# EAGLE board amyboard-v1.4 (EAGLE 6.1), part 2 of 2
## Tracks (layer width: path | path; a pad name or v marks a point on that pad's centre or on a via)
3V3_IN  (via drill 0.3)
  Top 0.61: D2.A 74.28,43.91 R59.1 74.3,45.99 v74.3,47.65 73.25,48.69 TP7.T | I2C_CONTROL.3 79.61,47.65 v79.43,47.65
  Top 0.813: Q3.2 74.96,44.59 D2.A
  Bottom 0.61: v79.43,47.65 v74.3,47.65
5V_IN
  Top 0.305: C34.2 C85.2 62.37,46.09 FB3.2 63.96,43.95 D14.A | C34.2 60.83,44.67 D3.A | C52.2 C34.2
  Top 0.406: R58.1 59.5,45.25 59.69,45.44
  Top 0.61: TP8.T 58.98,46.15 59.69,45.44
  pour Top: 59.28,46.43 64.77,46.43 64.77,42.83 60.76,42.83 59.46,44.12 59.28,44.3
12_IN  (via drill 0.3)
  Top 0.406: D1.A 68.58,40.82 | 68.58,40.82 D4.A | 68.1,39.83 69.14,39.83 | 69.62,40.29 69.62,39.83 69.14,39.83 | 69.14,39.83 v69.11,40.41 | 68.61,40.29 68.61,40.79 68.58,40.82 | 69.7,20.68 69,20.68 R57.1
  Top 0.61: v57.05,27.53 57.05,15.27 58.14,14.17 68.22,14.17 | P1.5 68.99,13.59 68.4,14.17 | 68.4,14.17 68.22,14.17 | 69.01,14.96 68.22,14.17 | 68.4,14.17 68.99,14.17
  Top 0.813: 69.62,40.29 68.61,40.29 | D1.A 68.83,41.58 69.77,41.58 69.22,41.02 68.58,41.02 | P1.5 68.99,14.17 P1.6 68.99,19.97 69.7,20.68 TP9.T
  Bottom 0.61: v69.11,40.41 61.72,40.41 60.81,39.5 60.81,37.52 55.93,32.64 55.93,28.65 v57.05,27.53
12V5_UNREG  (1 unrouted)
  Top 0.254: 59.33,29.57 59.82,30.05 60.25,29.62 61.09,29.62
  Top 0.406: U8.1 57.9,29.93 58.27,29.57 59.33,29.57 59.94,29.57 | 59.94,29.57 61.17,29.57 | U8.3 59.8,29.71 59.94,29.57
  Top 0.61: C18.1 61.87,28.98 R15.1
13.5V  (via drill 0.3)  (1 unrouted)
  Top 0.305: R15.2 61.32,31.27 61.29,31.29 | 62.28,31.29 62,31.57 62,31.85 62,31.88 62.08,31.95 | 62.47,31.41 62.45,31.41 62.18,31.67
  Top 0.406: v50.09,36.5 58.04,36.5 C29.1 58.84,35.7 R19.1 | R19.1 R16.1 61.06,33.64 D8.C | C20.2 59.94,34.76 R19.1 | C19.1 62.47,31.41 | 58.75,35.87 58.75,35.84 58.9,35.69 59.36,35.69 59.74,35.31 59.74,34.52 60.35,34.52 61.21,33.66 | 61.21,31.29 61.29,31.29 62.28,31.29 | 61.62,31.95 61.62,31.88 | 62,31.85 62,34.29 61.21,35.08 61.21,35.81 59.46,35.81 59.13,36.15 59.05,36.15 | 58.62,36.15 59.05,36.15 | 59.05,36.15 59.66,35.54 60.5,35.54 61.62,34.42 61.19,34.42 60.27,35.33 60.27,34.85 60.76,34.37 | U3.5 39.26,31.19 39.65,31.57 40.5,31.57 C26.2 40.58,31.62 v41.22,31.62
  Top 0.61: 61.21,33.66 61.21,31.29 | 62.18,31.95 62.08,31.95 61.62,31.95 | 61.62,31.88 61.82,31.67 62.18,31.67
  Bottom 0.406: v50.09,36.5 49.25,36.5 44.37,31.62 v41.22,31.62
+3V3  (via drill 0.3)  (3 unrouted)
  Top 0.254: C5.1 U1.22 27.33,26.57 26.42,27.48 | R54.1 R34.1 4.7,18.89 v4.7,19.43 | C33.2 R43.2 | 25.17,29.24 U1.36 25.42,29.05 | 25.17,29.24 25.17,31.17 24.8,31.54 | 25.4,28.7 24.99,29.11 | 24.99,29.11 24.99,29.36 | 24.99,29.36 24.99,30.48 | 24.33,31.34 24.77,31.34 24.99,31.12 24.99,30.48 | 26.42,27.48 26.34,27.56 25.53,27.56 24.99,28.09 24.99,29.11 | 24.99,29.36 25.16,29.2 | 25.16,29.2 25.2,29.16 25.2,28.17 25.68,27.69 26.34,27.69 26.36,27.71 26.36,27.81 | 26.36,27.81 26.31,27.76 25.65,27.76 25.43,27.99 25.43,28.5 | 24.99,30.48 v25.04,30.43 | C40.1 40.26,19.14 40.26,19.66 | C15.1 26.42,31.2 U1.34 26.42,27.48 | 39.27,22.63 39.32,22.68 40.66,22.68 40.82,22.53 40.82,19.33 40.39,18.9 39.42,18.9 39.19,19.13 | 40.56,21.01 40.64,21.08 v40.64,21.39 | 39.29,20.5 39.24,20.55 PCM5101.20 | v27.33,22.63 | 26.42,27.92 26.42,27.81 | 26.42,27.81 27.56,26.67 30.86,26.67 30.96,26.57 30.81,26.42 27.76,26.42 27.56,26.21 26.19,27.59 25.86,27.59 | 26.36,27.81 26.42,27.81 | 25.38,29.01 25.42,29.05 | 25.09,30.61 25.43,30.28 25.43,29.06 25.42,29.05 | 25.17,29.24 25.17,29.21 25.16,29.2 | C3.+ 38.75,19.16 38.99,18.92 | 86.21,35.21 86.41,35.21 C39.2
  Top 0.305: D12.4 R44.2 R42.2 R43.2 | 38.38,19.03 38.89,19.03 38.99,18.92 40.34,18.92 40.46,19.05 40.46,20.91 | 40.46,20.91 40.56,21.01 40.56,22.43 40.34,22.65 PCM5101.17 39.38,22.65 | 40.46,20.91 40.28,20.73 38.68,20.73 38.66,20.7 38.66,19.86 38.23,19.43 38.63,19.43 39.73,20.52 38.91,20.52 38.86,20.47 38.86,20.07 | 38.86,19.81 38.86,20.07 | 38.86,20.07 39.29,20.5 39.75,20.5 40.26,19.99 40.26,19.66 39.67,19.08 40.01,19.08 40.21,19.28
  Top 0.406: R35.1 14.02,15.04 | 14.02,15.04 C35.1 14.38,15.3 14.38,15.39 | U15.6 14.38,15.39 | 14.02,15.04 14.38,15.39 | v86.91,44.58 86.79,44.69 R41.2 82.49,44.69 L1.P$2 | R39.2 86.91,46.59 C27.1 87.4,46.84 89.08,48.51 92.43,48.51 93.04,49.12 93.04,51.77 91.77,53.04 89.72,53.04 R68.2 89.18,53 | D12.4 85.61,41.06 | 89.18,53 88.7,53 R69.2 | TP1.T 89.18,53.47 | 89.18,53.47 89.18,53 | 88.75,53.01 88.75,53.04 89.18,53.47 | 89.18,53.47 89.2,53.47 89.64,53.04
  Top 0.508: R40.2 v86.91,44.58 R39.2 | 97.16,33.78 97.16,34.71 R47.2
  Top 0.61: C37.2 96.84,35.03 R47.2 | C38.1 97.21,33.83 97.16,33.78 | R55.1 v84.18,33.78 84.78,33.78 | 84.18,42.49 82.25,42.49 82.02,42.72 L1.P$2 | 21.64,33.97 T1.4 v21.64,32.14 v21.64,32.13 | 84.78,33.78 84.99,33.78 C39.2 86.26,35.26 86.21,35.21 84.78,33.78 | U15.6 v14.38,22.1 | R49.2 77.75,20.07 76.02,21.79 HOST.1 | 39.19,19.13 39.19,19.51 40.11,20.42 40.11,19.84 39.47,19.2 40.13,19.2 40.54,19.61 40.54,20.7 40.72,20.88 | 40.72,20.88 40.72,22.38 | 40.72,20.88 40.72,19.48 40.34,19.1 | 27.33,26.57 v27.33,22.63
  Top 0.813: SD1.4 95.11,42.55 97.16,40.51 97.16,33.78 U2.2 | SD1.4 92.28,42.55 | Q3.3 84.18,42.49 | 84.18,42.49 85.61,41.06 86.21,40.46 86.21,35.21 | 79.35,42.5 80.09,43.23 83.82,43.23 83.82,42.85 84.18,42.5 | 84.18,42.49 84.18,42.5 | 84.18,42.5 84.18,44.15 84.81,44.78 86.39,44.78 86.82,44.35 86.82,46.46 86.67,46.31 86.67,46.05 85.65,45.04 83.82,45.04 83.03,44.25 83.84,44.25 84.45,44.86 86.11,44.86 86.59,45.34 | SD1.4 89.98,42.55 v89.97,42.57 | T1.1 T1.4
  Bottom 0.254: I2C_HOST.3 5.22,19.95 v4.7,19.43
  Bottom 0.61: v25.04,30.43 23.34,30.43 v21.64,32.13 | v84.18,33.78 84.18,23.9 82.6,22.33 HOST.1 74.45,22.33 73.2,21.08 53.65,21.08 53.16,20.6 41.43,20.6 39.4,22.63 v27.33,22.63 26.8,22.1 v14.38,22.1 10.31,22.1 8.15,19.94 5.8,19.94 I2C_HOST.3
  Bottom 0.813: v86.91,44.58 89.08,44.58 89.97,43.69 v89.97,42.57
-12.6V
  Top 0.61: D10.A 69.73,29.46 C31.2 67.61,29.46 67.41,29.67 | R17.2 67.41,29.67 | 67.41,29.67 C25.1
A3V3  (via drill 0.3)  (2 unrouted)
  Top 0.254: U5.8 2.41,21.54 v2.29,21.67 | C22.+ 42.78,26.31 v42.85,26.24 | U1.42 22.25,25.07 21.03,26.29 20.87,26.29 C11.1
  Top 0.305: R31.1 3.12,28.68 v3.57,29.12 4.01,29.57 4.01,30.2 4.06,30.25 4.06,30.18 4.04,30.15 4.04,31.27 4.01,31.29
  Top 0.406: 4.06,30.16 R20.2 | 42.85,25.15 42.85,24.77 43.33,25.25 43.26,25.25 42.88,25.63 | 42.85,25.15 42.85,28.66 C22.+ 42.67,28.21 42.67,21.13 43.11,20.7 PCM5101.1 45.79,20.7 C46.1 47.86,19.8 C45.+ 48.15,19.76 TP2.T | 42.85,25.15 42.95,25.25 PCM5101.8 47.23,25.25 C47.1 R13.2 R12.2 | 19.48,26.4 20.1,26.4 v20.17,26.47 | v61.01,24.69 61.01,24.14 R23.1 61,23.08 C54.1 61.02,23.1 U10.1
  Top 0.61: C11.1 19.48,26.4 C12.+
  Bottom 0.406: 20.17,26.65 v20.17,26.47 19.99,26.65 | 20.17,26.65 20.4,26.65 | 20.4,26.65 42.44,26.65 v42.85,26.24 44.4,24.69 v61.01,24.69 | 3.94,26.65 3.67,26.65 3.57,26.75 v3.57,29.12 3.57,22.95 v2.29,21.67 | 3.94,26.65 19.94,26.65 | 19.94,26.65 19.99,26.65 | 19.99,26.65 20.17,26.65 | 3.58,27 3.94,26.65 | 3.94,26.65 3.58,26.29 | 20.4,26.65 20.17,26.42 19.94,26.65
A5V  (via drill 0.3)
  Top 0.254: C16.+ 21.96,21.21 C13.1 22.52,23.07 U1.46 v26.04,23.06
  Top 0.61: U9.1 TP3.T C53.1 v72.64,21.9
  Bottom 0.254: v72.64,21.9 53.34,21.9 52.78,21.34 41.81,21.34 39.83,23.32 26.29,23.32 v26.04,23.06
A12V  (via drill 0.3)
  Top 0.406: U4.4 v49.07,31.85 | C32.1 57.28,33.38 | 57.28,33.38 57.8,33.38 U8.5 | v57.3,32.72 57.3,33.35 57.28,33.38 | 56.34,33.4 56.62,33.4 v57.3,32.72 | v57.3,32.72 57.58,33 57.96,33
  Top 0.61: TP4.T 45.85,31.85 U4.4 | U10.3 66.27,23.88 66.27,25.58 | 66.27,25.58 v66.27,26.44 v66.28,26.44 U9.3 | 67.54,26.37 67.54,26.01 66.7,26.01 66.27,25.58
  Bottom 0.406: v49.07,31.85 49.07,28.93 51.59,26.42 57.45,26.42 | 57.45,26.42 57.99,26.42 | 57.99,26.42 58.52,26.42 | 58.52,26.42 66.24,26.42 v66.27,26.44 | v57.3,32.72 57.3,28.65 57.99,27.97 57.99,26.95 | 57.99,26.95 57.99,26.42 | 57.45,26.42 57.99,26.95 | 57.99,26.95 58.52,26.42
A-12V
  Top 0.406: 56.79,30.35 56.74,30.4 56.74,30.43 TP5.T 56.6,30.34 56.43,30.34 | 57.93,28.81 U7.5 57.93,28.84 56.43,30.34 | U4.11 53.72,31.85 54.28,31.29 C28.1 55.47,31.29 56.43,30.34
ADC1  (via drill 0.3)  (1 unrouted)
  Top 0.254: 2.59,31.29 R6.1 2.79,31.66 v2.79,31.8 2.79,31.5 2.59,31.29 | 2.59,31.29 C10.1 R8.2 | R8.2 2.06,32.35 R5.1 | 2.25,32.16 R8.2 | 1.91,24.64 1.91,25.81 v2.02,25.92
  Bottom 0.254: v2.79,31.8 2.79,26.21 2.5,25.92 v2.02,25.92
ADC2
  Top 0.254: R20.1 R21.2 C9.1 R7.1 2.07,27.97 1.55,27.97 1.41,27.83 U5.5
AMY_FOLLOWER_SCL  (via drill 0.3)
  Top 0.406: v93.37,32.97 93.37,32.02 U2.5 | I2C_CONTROL.1 76.12,50.65 77.17,51.69 87.2,51.69 87.66,51.69 | 87.66,51.69 v87.71,51.74 | R69.1 88.23,51.69 87.66,51.69
  Bottom 0.406: v93.37,32.97 93.88,33.48 93.88,45.57 v87.71,51.74
AMY_FOLLOWER_SDA  (via drill 0.3)  (1 unrouted)
  Top 0.406: U2.4 v94.62,32.97 v94.61,32.97 | I2C_CONTROL.2 78.12,50.31 78.84,51.03 v89.56,51.03 | R68.1 89.69,51.13 89.56,51
  Bottom 0.406: v94.61,32.97 94.61,45.97 v89.56,51.03
AMYIN  (via drill 0.3)
  Top 0.254: U2.17 79.43,27.69 79.3,27.56 v79.3,26.59 | U1.17 34.25,24.07 v34.37,23.95
  Bottom 0.254: v34.37,23.95 40.06,23.95 42.16,21.84 52.4,21.84 53.06,22.51 73.53,22.51 77.62,26.59 v79.3,26.59
AMYOUT  (via drill 0.3)  (1 unrouted)
  Top 0.254: U1.10 29.92,22.93 v30.96,23.98 | v82.58,27.18 88.24,27.18 92.08,31.01 U2.6 | PCM5101.14 40.12,24.6 40.13,24.59 v40.28,24.59
  Top 0.305: R33.2 92.04,31.89 92.13,31.8 92.13,32 92.08,32.06
  Bottom 0.254: 31.09,24.11 v30.96,23.98 31.57,24.59 v40.28,24.59 42.52,22.35 52.17,22.35 52.83,23.01 73.18,23.01 77.34,27.18 v82.58,27.18
BCLK  (via drill 0.3)
  Top 0.254: U1.19 | U1.19 38.15,25.07 38.33,25.25 PCM5101.13 40.34,25.25 v41.1,26.01 | U1.8 28.92,23.56 30.43,25.07 U1.19 | U2.12 84.46,30.91 84.23,30.68 v82.6,30.68
  Bottom 0.254: v41.1,26.01 42.16,26.01 44.09,24.08 72.57,24.08 77.42,28.93 82.5,28.93 82.8,29.24 82.8,30.48 v82.6,30.68
CV_OUT1  (via drill 0.3)
  Top 0.406: CV_OUT1.LEFT/TIP 24.99,48.39 v30.48,42.9 | R61.1 43.52,35.74 v43.18,35.74
  Bottom 0.406: v30.48,42.9 30.5,42.9 37.21,35.74 v43.18,35.74
CV_OUT2  (via drill 0.3)  (1 unrouted)
  Top 0.406: v44.02,29.34 44.7,29.34 44.86,29.19
  Bottom 0.406: CV_OUT2.LEFT/TIP 13.99,50.12 15.11,49 24.43,49 29.62,43.82 29.62,39.57 28.96,38.91 28.96,34.75 34.37,29.34 v44.02,29.34
DTR
  Top 0.305: HOST.5 76.02,11.3 76.86,10.47 79.78,10.47 80.03,10.72 80.03,12.14 80.29,12.4 81.04,12.4 Q5.2 | 80.85,12.2 Q5.2 | Q5.2 81.09,12.45 R48.2
ENABLE
  Top 0.406: U6.4 62.3,37.87 63.25,38.81 R14.2
GND  (via drill 0.3)  (1 unrouted)
  Top 0.254: USB.GND2 63.73,50.14 62.33,48.74 C85.1 | 35.2,25.81 35.05,25.65 33.68,25.65 33.27,26.07 U1.21 | 35.2,25.81 35.2,26.57 35.23,26.59 35.2,26.59 | 39.21,25.93 PCM5101.12 | 39.21,25.93 39.21,26.51 PCM5101.11 39.24,27.61 39.05,27.8 38.58,28.27 | 99.36,10.06 99.52,10.06 99.54,10.03 99.57,10.03 98.81,10.8 98.81,11.56 | RST.4 92.61,10.57 RST.1 | U1.26 30.4,29.01 30.4,30.2 | U1.23 33.57,27.07 33.76,27.26 35.13,27.26 35.26,27.13 35.26,26.58 | 39.21,25.93 35.33,25.93 35.2,25.81 | 38.12,21.29 38.18,21.34 39.24,21.34 | U1.45 24.94,23.57 v25.98,24.61 25.98,25.58 | 25.98,25.58 25.98,26.65 25.58,27.05 24,27.05 U1.38 | 21.04,27.1 22,27.1 22,26.52 22.95,25.57 U1.41 25.97,25.57 25.98,25.58 | C17.1 19.62,25.21 v19.53,25.12 18.07,25.12 R4.2 | U5.3 2.41,23.09 2.13,22.81 | C32.2 58.73,31.85 58.88,32 | 41.96,9.12 42.04,9.12 v42.27,9.35 | 1.7,21.08 1.7,20.7 | 1.7,20.7 1.7,19.69 | U5.7 1.91,20.49 1.7,20.7 | 36.45,23.27 37.54,23.27 37.49,23.22 C41.1 | 57.91,27.05 58.83,27.97 | 59.05,27.92 59.05,27.79 59.69,27.15 | 32.38,27.08 31.42,27.08 31.34,27.15 30.35,27.15 30.18,27.33 30.18,28.83
  Top 0.305: R33.1 91.15,35.27 SD1.G1 | PCM5101.9 PCM5101.10 | 39.98,28.73 39.05,27.8 | 38.58,28.27 38.58,28.7 38.12,29.16 38.12,29.75 U3.4 | U3.4 U3.3 | U3.4 37.9,30.25 v37.9,31.14 37.9,31.95 | 37.9,31.95 U3.EP 35.87,32.59 v35.56,32.28 | U3.6 39.26,33.32 37.9,31.95 | PCM5101.3 44.22,22 | C48.1 50.65,22.53 50.77,22.66 50.77,23.36 C50.1
  Top 0.406: U6.2 65.85,36.58 R18.2 | 31.41,13.62 R67.2 | C15.2 26.26,32.67 v26.31,32.72 | 30.15,28.45 v30.15,30.23 | 44.07,26.24 46.1,26.24 | 38.25,26.19 40.13,26.19 | 48.16,12.12 48.16,11.86 48.82,11.2
  Top 0.61: R25.1 R26.1 R29.1 R30.1 | C38.2 98.86,35.01 C37.1 100.33,35.03 SD1.G2 | C36.1 94.18,33.96 v92.66,35.48 | v92.66,35.48 91.81,35.48 SD1.G1 | v92.66,35.48 92.66,36.96 v92.81,36.96 | 19.2,20.07 19.2,21.74 19.28,21.82 20.42,21.82
  Top 0.813: C38.2 98.86,32.42 U2.1
  Bottom 0.254: 83.54,33.43 83.54,32.67 82.45,31.57 v80.87,31.57
  Bottom 0.406: v64.36,31.52 63.48,31.52 63.48,32.41 63.45,32.41 63.45,32.44
  Bottom 0.813: LINE_IN.GND 53.21,37.63
  Bottom 1.27: 53.45,37.87 LINE_IN.GND
  other vias: 97,11.05 41.63,42.39 46.58,37.47 44.45,30.28 58.88,32.74 72.19,13.89 86.94,19.58 78.74,41.48 90.5,22.89 88.95,25.93 94.87,25.58 92.53,21.64 88.6,34.11 88.87,19.61 94.92,27.41 72.26,45.16 85.98,21.57 91.29,21.82 89.31,23.78 100.3,42.83 72.26,44.4 67.34,36.45 87.4,21.44 99.09,49.33 40.94,43.54 90.47,33.94 89.89,21.26 94.18,29.92 92.94,29.97 89.08,22.05 17.7,30.86 23.7,35.21 18.87,30.38 20.29,30.56 9.17,11.89 24.46,10.39 8.03,11.48 16.51,11.84 2.57,14.99 16.54,13.11 13.41,11.02 9.86,9.65 10.39,10.97 16.33,10.42 17.14,15.62 4.32,9.42 20.27,19.56 22.3,14.83 22.58,12.52 22.58,11.13 18.8,9.63 12.34,10.01 13.18,19.2 12.4,20.17 1.27,13.67 1.88,18.75 15.32,19.81 13.26,12.27 22.28,13.44 28.45,9.4 38.05,20.37 43.13,34.52 39.19,28.53 45.9,38.36 47.29,38.05 47.35,45.19 48.49,45.52 48.54,46.61 13.74,46.23 47.24,47.52 46.25,46.66 46.18,44.5 46.23,48.57 31.34,52.93 42.34,51.56 42.06,49.89 44.3,50.9 20.65,51.16 25.88,55.37 84.3,9.6 86.41,9.58 83.06,11.43 84.07,11.41 85.12,11.48 82.5,19.58 69.98,54.28 74.3,15.55 74.22,9.4 83.62,9.22 85.22,9.3 97.49,16.59 98.2,20.88 58.85,31.95 97.74,18.04 100.23,38.2 75.13,16.1 84.56,20.52 94.39,23.55 75.82,38.38 95.86,37.11 97.21,42.52 85.42,15.83 100.89,53.52 67.67,19.31 92.35,54.15 43.76,9.32 102.95,51.79 97.28,54.66 94.77,54.59 101.32,55.47 72.92,16.79 98.65,42.77 67.36,17.81 65.23,11.35 105.33,52.6 55.04,11.3 55.98,9.7 97.92,52.3 62.61,11.48 60.35,17.37 61.29,15.34 54.03,9.78 57.25,11.46 57.33,10.01 60.07,10.47 31.9,9.55 96.7,49.18 56.39,10.62 48.16,11.94 72.85,9.27 70.97,9.88 62.76,13.01 91.03,11.96 60.1,11.41 72.54,54.69 91.21,28.2 94.59,51.92 6.96,9.58 3.43,13.89 8.31,14.5 5.66,10.64 9.17,13.41 0.71,13.11 0.69,15.29 20.14,29.72 38.46,32.56 24.69,36.35 44.53,40.26 26.77,34.72 32.11,30.2 35.13,36.58 0.84,51.69 1.07,49.18 33.38,49.79 0.84,47.42 33.76,51.39 0.84,44.86 36.5,55.65 0.84,41.17 30.25,52.3 1.93,44.12 30.84,49.91 2.29,48.92 2.64,51.31 12.17,49.56 0.79,36.96 6.12,45.19 0.76,33.45 2.26,38.79 7.75,32.44 2.95,41.07 3.1,42.98 3.02,45.21 3.1,47.12 3.84,49 4.06,55.75 6.73,55.8 5.28,54.18 15.32,55.3 7.72,50.9 10.21,53.19 8.89,52.1 52.07,41.63 35.23,33.66 34.37,48.49 34.34,40.31 44.3,41.5 38.63,37.8 39.75,37.82 43.21,40.36 42.82,33.76 55.24,49.79 31.78,43.69 34.39,44.35 45.26,47.68 44.58,42.65 43.05,43.13 21.97,49.99 38.99,45.19 37.54,46.81 35.15,47.25 39.73,46.43 37.47,48.69 35.81,45.37 33.4,43.03 50.22,38.23 9.7,24.18 15.52,24.23 13.34,20.04 17.3,19.99 1.07,39.37 6.32,31.12 13.26,35.64 6.48,33.71 0.74,22.66 1.63,22.45 0.66,19.69 9.04,29.21 5.21,32.54 8.36,35.79 15.24,45.31 21.95,42.6 12.4,38.86 42.09,11.66 24.23,46.03 27.79,47.14 21.92,40.97 21.06,39.93 33.3,31.67 32.13,33.53 34.06,38.13 19.81,31.17 34.65,31.04 36.45,33.02 16.33,18.67 16.13,23.39 23.42,11.89 38.73,33.45 22.86,9.93 52.5,9.5 52.04,11.3 54.1,10.85 47.57,9.65 47.29,17.63 42.88,17.45 50.47,17.45 47.14,13.84 44.32,13.87 93.95,11.38 97.76,12.75 101.22,13.06 100.97,11.15 101.42,9.53 105.05,13.13 103.23,13.49 99.49,12.93 98.83,16.61 98.6,19.05 97.33,19.41 98.96,29.47 98.91,27.36 98.96,25.45 98.98,23.55 98.98,21.72 98.15,47.83 102.16,43.49 104.47,48.52 103.78,42.47 103.78,39.42 104.22,45.59 104.47,34.52 101.37,34.82 99.44,39.6 95.66,39.22 89.28,40.34 87.15,42.04 88.01,42.11 97.49,24.97 102.39,33.58 72.14,39.96 41.05,9.73 40.77,11.02 79.73,31.83 77.62,41.17 99.19,37.52 73.05,35.56 100.99,49.02 101.75,41.05 75.67,33.33 96.72,45.11 100.13,45.39 87.48,54.31 93.98,55.12 85.75,54.31 83.13,54.64 80.87,54.33 75.11,54.76 68.48,55.02 65.66,55.07 68.43,51.94 65.53,52.43 60.12,55.6 57.58,55.7 60.53,51.54 60.86,49.38 54.33,50.83 52.83,50.83 38.79,55.45 73.86,49.68 72.75,50.19 70.23,48.11 74.07,51.08 58.45,47.63 98.35,45.42 14.15,37.97 57.15,44.71 65.71,45.87 67.44,10.95 69.82,36.12 84.18,38.41 94.44,49.1 95.89,47.58 92.35,39.75 92.28,40.95 101.02,33.17 74.47,34.98 90.2,27.08 90.4,25.55 93.57,27.38 92.3,26.06 91.72,23.85 93.47,25.15 81.64,49.79 86.61,55.6 75.31,50.5 100.13,47.58 79.15,18.82 78.61,19.18 65.15,13.03 90.93,10.77 5.51,35.03 3.25,33.22 10.64,13.87 5.51,28.35 41.99,34.11 36.7,37.64 41.61,34.93 33.2,29.47 37.44,28.53 36.73,25.99 62.56,16.43 58.29,31.95 62.61,17.63 60.48,12.93 62.43,15.39 65.05,16.87 62.76,10.57 65.1,15.42 65.23,10.31 67.41,16.92 70.97,11.15 70.1,14.58 71.07,15.8 36.35,47.85 73.56,14.43 71.88,17.55 63.37,33.35 72.97,11.28 66.78,15.47 61.57,28.22 32.66,39.24 79.1,13.69 74.32,11.02 67.34,13.03 73.89,13.18 73.13,12.55 72.14,11.96 85.17,19.53 82.17,11.43 87.58,9.83 87.43,12.62 92.94,12.52 96.93,17.5 104.83,50.17 76.94,24.23 77.95,24.49 77.83,25.58 78.92,25.55 79.07,24.56 78.94,23.72 90.53,20.24 82.98,15.85 60.22,15.42 74.04,34.09 77.77,23.55 69.82,28.25 72.29,28.12 77.88,32.82 39.7,12.14 78.33,31.9 89.41,15.83 79.2,32.87 92.3,28.91 102.59,48.26 83.24,28.2 103.68,37.44 91.03,54.97 83.31,49.1 78.05,54.53 89.03,36.78 86.08,20.37 43.33,10.72 74.42,19.46 36.07,10.16 71.12,36.2 63.32,34.27 65.13,19.38 31.67,39.8 72.42,10.16 70.99,16.97 58.85,33.5 93.01,19.99 41.45,13.87 48.9,17.78 73.94,17.6 57.18,12.96 63.63,15.32 60.3,16.21 46.61,27.03 59.64,31.98 97.56,28.2 88.7,28.86 88.7,30.28 89.69,30 82.25,28.07 90.7,30.68 39.6,17.55 33.27,20.98 37.24,20.12 65.23,17.65 60.1,19.33 3.78,14.96 25.17,11.41 26.29,10.21 11.38,11.76 15.11,11.43 23.34,13.89 23.93,13.16 25.43,25.55 26.47,25.91 26.01,25.45 25.5,23.88 30.94,19.31 32.05,17.37 36.07,25.99 37.49,25.99 38.4,28.55 40.06,28.53 41.53,30.23 41.45,30.94 43.64,30.94 42.24,30.94 40.08,32.41 39.27,34.01 36.22,31.42 34.06,33.4 34.09,31.93 31.04,35.46 31.9,29.52 34.77,32.54 37.39,11.1 43.89,17.5 43.38,23.09 41.4,24.64 33.15,16.87 36.78,32.26 22.45,25.93 26.49,25.1 20.27,25.55 18.69,25.3 18.29,20.5 17.04,24.13 12.6,34.32 19.66,32.39 18.21,31.8 15.82,29.72 4.9,25.17 20.73,31.78 37.64,31.98 8.05,21.29 8.15,24.13 13.49,33.43 8.76,22.91 11.05,24.39 9.96,20.45 11.68,19.31 5.99,13.64 1.12,17.55 0.69,25.53 0.66,28.14 9.8,40.06 9.63,43 16.38,46.28 26.19,44.76 19.13,41.45 17.96,37.36 24.28,44.37 37.72,17.88 40.36,17.35 47.5,27.1 65.05,51.72 63.42,35.41 63.53,36.6 63.47,32.44 67.31,28.04 75.01,35.48 75.39,32.49 73.28,34.65 71.09,28.14 73.43,28.14 75.77,36.93 74.32,32.94 72.92,33.48 66.83,31.62 72.16,43.38 76.48,32.89 68,31.57 58.88,28.78 46.1,11.25 68.55,28.09 39.57,9.88 55.27,19.31 38.25,12.07 62.61,19.36 48.59,9.42 49.2,11.23 49.43,10.06 45.26,9.45 42.24,10.75 45.21,17.58 26.8,17.63 46.13,17.55 41.71,17.6 64.54,30.71 41.88,24.13 39.27,13.87 78.31,35.87 78.36,34.82 78.84,30.99 72.26,42.52 16.64,30.43 14.5,12.24 14.53,9.96 7.34,12.8 5.36,12.57 2.16,15.93 11,18.31 12.6,18.29 11,15.98 12.65,16.13 19.68,19.89 7.67,16.94 9.47,14.66 15.93,20.55 10.59,23.39 16.56,19.58 16.36,24.97 4.78,21.29 6.93,23.6 6.25,22.68 6.76,21.29 1.57,23.34 2.77,23.39 6.07,25.88 4.29,25.88 4.24,24.16 10.97,29.13 7.32,29.19 6.58,36.68 11,35.71 16.33,38.99 11.86,42.55 9.47,50.39 12.83,55.37 17.7,55.3 22.43,52.55 19.28,52.66 19.15,50.27 28.24,55.4 23.7,55.35 26.26,53.82 34.44,55.53 55.78,50.85 59.49,53.14 65.53,44.6 94.82,13.21 96.14,13.01 94.34,28.7 67.08,54.36 52.1,50.09 50.95,45.54 50.95,46.76 50.9,47.55 42.93,30.13 53.49,49.73 51.05,37.9 6.1,47.32 44.7,10.42 34.42,16.82 50.01,17.78 47.62,10.69 90.98,18.8 97.21,29.59 97.59,26.65 94.34,22 97.38,22.84 79.68,14.76 86.18,23.29 85.8,49.91 85.85,48.24 79.58,49.66 83.69,47.78 83.13,50.14 75.67,51.69 87.1,48.49 83.95,46.56 89.97,46.86 90.63,51.89 91.85,51.97 91.24,51.59 89.1,47.09 92.23,49.73 36.98,20.65 35.99,12.07 34.14,13.89 31.39,11.58 25.27,36.7 24.31,35.26 35.05,19.61 35.05,17.76 16.41,17.5 18.21,15.93 20.22,15.93 19.15,16.46 20.73,20.12 50.88,12.32 46.84,11.69 55.09,14.25 55.42,17.65 55.37,16.69 55.35,15.34 32.49,13.87 29.92,35.43 28.02,35.61 26.97,35.56 45.09,37.75 45.54,27.23 44.65,27.28 81.23,11.48 60.76,27.97 60.99,28.53 44.78,11.69 68.45,36.22 64.67,29.8 64.01,28.14 66.75,30.81 65.33,29.24 67.92,15.27 58.85,15.09 50.95,13.87 70.56,19.41 75.51,10.82 32.77,9.5 37.62,9.68 29.39,9.78 20.95,9.53 16.92,9.65 36.63,13.87 31.47,16.69 27.43,16.69 28.4,16.56 29.64,17.55 32.46,32.69 31.93,35.05 26.82,32.97 8,30.1 15.44,18.67 15.95,15.93 12.95,32.44 21.34,15.65 19,15.32 16.76,14.33 31.45,12.42 31.29,10.36
  pour Bottom (isolate 0.203, rank 6): -10,68.61 120,68.61 120,-1.39 -10,-1.39
  pour Top (isolate 0.203, rank 6): -11,69.61 121,69.61 121,-2.39 -11,-2.39
I2C_SCL  (via drill 0.3)
  Top 0.254: 30.92,28.3 U1.25 30.96,29.04 | 30.92,28.3 v30.92,27.74 v30.91,27.74 | v81.92,30.1 84.91,30.1 85.72,30.91 U2.11 | v3.53,19.41 3.53,19.17 3.81,18.89 R34.2 3.41,19.26 U5.10 3.41,21.27 7.62,25.48 v7.62,27.74 | U3.1 35.26,28.99 34.95,28.68 31.3,28.68 30.92,28.3 | 35.23,29.67 35.23,29.26 34.85,28.88 31.45,28.88 | 31.27,28.88 30.96,28.58 30.96,29.04 | 30.96,29.31 30.96,29.19 | 30.96,29.19 31.27,28.88 | 31.27,28.88 31.45,28.88 | 31.45,28.88 30.96,29.36 | 30.96,29.19 30.96,29.04
  Bottom 0.254: v7.62,27.74 v30.91,27.74 30.99,27.81 42.93,27.81 44.91,25.83 72.75,25.83 77.01,30.1 v81.92,30.1 | I2C_HOST.1 4.07,15.95 3.12,16.89 3.12,19 v3.53,19.41
I2C_SDA  (via drill 0.3)
  Top 0.254: v82.2,29.52 85.7,29.52 87,30.81 U2.10 | v3.79,17.3 3.8,17.31 R54.2 3.2,17.78 2.91,18.07 U5.9 2.91,21.56 7,25.64 v7,27.31 | U1.24 32.85,28.07 35.84,28.07 | 35.84,28.07 36.26,28.07 | 32.64,27.56 32.99,27.92 35.89,27.92 36.25,27.56 | 36.25,27.56 36.25,27.53 | 36.25,27.66 36.25,28.53 | 36.25,28.65 36.25,28.53 | 36.25,28.53 35.76,28.04 | 36.25,27.56 36.25,27.66 | 36.25,27.66 35.84,28.07
  Top 0.406: U3.2 36.26,28.07 v36.26,27.23
  Bottom 0.254: v82.2,29.52 77.17,29.52 72.97,25.32 44.65,25.32 42.75,27.23 v36.26,27.23 36.19,27.15 7.16,27.15 v7,27.31 | I2C_HOST.2 4.44,17.95 v3.79,17.3
IO0
  Top 0.305: Q5.3 79.05,12.55 80.99,14.49 U2.27 81.92,13.87 82.42,13.36 93.58,13.36 BOOT.2
  Top 0.406: Q5.3 77.76,11.48 R49.1
IO19  (via drill 0.3)
  Top 0.406: R45.2 v67.54,46.69 | U2.13 83.19,32.64 v82.86,32.97
  Bottom 0.406: v67.54,46.69 79.38,46.69 82.65,43.41 82.65,33.17 v82.86,32.97
IO20  (via drill 0.3)
  Top 0.406: R46.2 v66.5,46.69 | U2.14 v81.92,32.97
  Bottom 0.406: v66.5,46.69 67.16,46.03 78.89,46.03 81.92,43 v81.92,32.97
LIN  (via drill 0.3)
  Top 0.406: v53.59,27.15 53.59,15.75 v53.09,15.24 | R2.2 C59.2 18.35,17.95 D7.2 v17.5,17.96
  Bottom 0.406: LINE_IN.LEFT/TIP 47.14,41.76 47.14,43.84 47.45,44.15 50.8,44.15 51.38,43.56 53.19,43.56 57.91,38.73 57.99,37.19 57.99,37.04 56.03,35.08 54.91,35.08 53.59,33.76 v53.59,27.15 | v53.09,15.24 25.2,15.24 22.48,17.96 v17.5,17.96
LINX
  Top 0.254: U1.47 23.05,22.57 22.76,22.28 22.76,19.82 C43.+
LINX_ADC
  Top 0.406: C65.2 R73.1
LOUT  (via drill 0.3)  (1 unrouted)
  Top 0.406: R63.1 55.44,27.57 v55.04,27.18
  Bottom 0.406: 59.82,48.37 59.82,37.77 56.16,34.11 55.98,33.94 55.04,33 v55.04,27.18 | LINE_OUT.LEFT/TIP 46.99,50.52 48.56,49 59.18,49 59.77,48.36
LOUT_2V  (via drill 0.3)
  Top 0.305: R51.1 49.28,23.5 | 49.28,23.5 49.77,23.5 C50.2 | v49.2,23.47 49.2,23.42 49.28,23.5 | U4.10 51.49,30.58 51.13,30.23 51.13,25.71 51.54,25.3 v51.54,23.47
  Bottom 0.254: v49.2,23.47 v51.54,23.47
LRC  (via drill 0.3)
  Top 0.254: PCM5101.15 38.41,23.95 37.79,24.57 U1.18 30.66,24.56 29.42,23.32 U1.9 v29.42,19.21
  Top 0.305: U2.38 95.89,15.31 93.32,17.88 v84.2,17.88 | v29.41,19.2 v29.42,19.21
  Bottom 0.305: v84.2,17.88 77.78,17.88 77.11,18.54 30.07,18.54 v29.41,19.2
MCLK  (via drill 0.3)  (1 unrouted)
  Top 0.254: U1.7 28.42,24.38 v29.44,25.4 29.62,25.58 U1.20 32.38,25.55 | U2.15 80.01,30.23 79.43,29.64 v79.43,28.35
  Bottom 0.254: v79.43,28.35 77.67,28.35 72.85,23.52 52.6,23.52 51.94,22.86 44.55,22.86 42.01,25.4 v29.44,25.4
MIDI_A_OUT
  Top 0.305: U2.22 R37.2
MIDI_B_OUT
  Top 0.406: U2.8 R38.2
MIDI_IN  (via drill 0.3)
  Top 0.406: R35.2 10.34,15.04 9.3,16.08 U15.4 9.3,18.72 v11.28,20.7 | U2.23 v79.43,20.07
  Bottom 0.406: v79.43,20.07 77.75,20.07 76.73,21.08 74.65,21.08 73.79,20.22 54.1,20.22 53.62,19.74 41.05,19.74 38.99,21.79 27.79,21.79 27.25,21.26 11.84,21.26 v11.28,20.7
N$1  (1 unrouted)
  Top 0.254: U1.37 23.99,29.77 C1.1 | 23.16,30.38 23.8,29.74 23.8,27.64 23.88,27.56 24.16,27.56 24.21,27.61 24.21,29.85 23.55,30.51 23.29,30.51
N$2
  Top 0.254: C4.2 34.96,21.95 R3.1
N$3
  Top 0.254: U1.15 C4.1
N$4
  Top 0.406: R66.1 C63.- 30.19,10.64 1-10VPP.1 27.76,10.64 21.97,16.43 C43.- 20.57,17.03 R2.1
N$5
  Top 0.406: R67.1 30.47,12.37 C64.- 30.01,11.91 1-10VPP.2 27.81,11.91 25.54,14.19 R1.1 24.22,16.54 C44.-
N$6
  Top 0.254: U1.44 22.34,24.07 21.59,23.32 20.1,23.32 | 20.1,23.32 C7.1 | C8.+ 18.79,23.32 20.1,23.32
N$7
  Top 0.254: U1.43 21.9,24.57 21.64,24.31 21.02,24.31 C17.2 19.96,24.32 C6.2
N$8
  Top 0.254: C6.1 18,24.33 R4.1
N$13  (via drill 0.3)
  Top 0.406: R7.2 v2.08,26.62
  Bottom 0.406: v2.08,26.62 2.08,34.09 9.6,41.61 CV_IN2.LEFT/TIP
N$15  (via drill 0.3)
  Top 0.406: C21.2 U7.2 v58.88,27.13 | R17.1 66.53,29.15 v66.12,28.73
  Bottom 0.406: v58.88,27.13 64.52,27.13 v66.12,28.73
N$16
  Top 0.406: MB14F.DCMINUS 10.26,31.47 11.93,29.8 D13.+ 11.93,26.21 U15.2
N$18
  Top 0.305: U3.8 37.26,36.58 37.77,37.08 40.23,37.08 40.84,36.48 40.84,33.81 41.53,33.12 44.12,33.12 | 44.12,33.12 U4.3 | C23.2 44.12,33.12
N$19
  Top 0.406: R5.2 2.35,34.35 12.22,44.22 18.01,44.22 20.62,41.61 CV_IN1.LEFT/TIP
N$20
  Top 0.305: U3.7 38.26,36.18 38.51,36.42 39.78,36.42 40.13,36.07 40.13,33.38 41.05,32.46 42.93,32.46 | 42.93,32.46 43.87,32.46 45.74,30.58 U4.5 | C24.2 42.9,32.44 42.93,32.46
N$21
  Top 0.254: 64.57,35.71 64.65,35.63 U6.1
  Top 0.406: U6.1 65.45,34.88 D8.A 66.19,32.56 R24.2 69.55,32.58 L3.P$2 | 64.41,35.66 64.41,32.31 69.67,32.31 69.67,34.65 69.49,34.82 67.39,34.82 66.5,35.71 64.57,35.71 64.92,35.36 66.34,35.36 67.23,34.47 67.44,34.47 68.05,33.86 69.16,33.86 69.22,33.81 69.22,32.89
  Top 1.016: 69.22,32.89 68.89,33.22 66.52,33.22 67.03,33.73 67.03,34.14 66.22,34.95 64.77,34.95 65.66,34.06 66.5,34.06
N$22
  Top 0.61: C42.+ 34.73,34.76 U3.10
N$23  (via drill 0.3)
  Top 0.61: Q3.1 77.29,43.59 76.4,43.59 76.02,43.21 76.02,42.55 | 76.02,42.55 74.3,40.82 D4.C | 76.02,42.55 76.02,41.31 R11.2 v75.4,41.3 75.39,41.3 74.73,40.64 74.73,40.69 75.79,41.76
  Top 0.635: D3.C v61.39,41.35
  Top 1.27: D5.A 73.99,37.97 73.99,40.55 D4.C
  Bottom 0.635: v61.39,41.35 v75.4,41.3
N$24  (via drill 0.3)
  Top 0.61: D5.C 78.05,37.98 C106.1 v78.92,40.03 | v81,35.89 U12.5 82.56,35.89 R60.1
  Bottom 0.61: v81,35.89 81,37.95 v78.92,40.03
N$25
  Top 0.61: U12.6 81.48,37.1 C55.2
  Top 0.813: C55.2 81.48,39.98 L1.P$1
N$26  (1 unrouted)
  Top 0.406: 44.86,28.32 44.87,28.31 R10.1 47.37,28.31 U4.7
N$27
  Top 0.61: R24.1 71.48,32.56 C30.1
N$28
  Top 0.406: U6.5 61.07,36.58 R16.2
N$29
  Top 0.813: C30.2 74.5,31.22 76.05,31.22 76.52,30.74 D9.A
  Top 1.016: D10.C 74.67,30.35 75.84,30.35 76.23,30.74 D9.A
N$30
  Top 0.406: U7.3 59.83,24.41 R23.2
N$31
  Top 0.305: R13.1 48.59,26.72 49.12,27.26 49.12,28.98 48.79,29.31 U4.6
  Top 0.406: U4.6 45.91,29.31 R10.2
N$32
  Top 0.406: R61.2 R27.1 45.86,35.66 U4.1
N$33
  Top 0.305: R12.1 49.81,26.66 49.81,33.63 49.05,34.39 U4.2
  Top 0.406: U4.2 45.96,34.39 R27.2
N$34
  Top 0.305: R48.1 85.18,12.45 Q2.1
N$35
  Top 0.406: 1-10VPP.5 R30.2
N$36
  Top 0.406: 1-10VPP.6 R29.2
N$37
  Top 0.305: Q5.1 R9.1
N$38
  Top 0.279: USB.A5 68.2,48.45 R53.1
N$39
  Top 0.279: USB.B5 65.2,48.4
  Top 0.305: 65.2,48.4 R52.1
N$40
  Top 0.254: 19.16,10.64 R25.2
  Top 0.406: 1-10VPP.8 19.16,10.64
N$41
  Top 0.406: 1-10VPP.7 R26.2
N$42  (via drill 0.3)
  Top 0.305: 69.39,50.37 USB.VBUS1
  Top 0.559: USB.VBUS2 64.5,49.47
  Top 0.61: 64.5,49.47 v64.21,49.18 63.96,48.92 FB3.1 | v69.39,49.18 69.39,50.37
  Bottom 0.61: v64.21,49.18 v69.39,49.18
N$43
  Top 0.254: U5.2 2.91,26.85 R31.2
N$44  (via drill 0.3)
  Top 0.406: 1-10VPP.3 v29.44,13.18 | v55.88,13.18 56.31,13.62 56.31,29.49 55.82,29.99 C57.1 R22.2 53.98,29.97 53.31,29.31 U4.9
  Bottom 0.406: v29.44,13.18 v55.88,13.18
N$45  (via drill 0.3)
  Top 0.254: C58.1 55.61,34.37 v55.27,34.37
  Top 0.406: 1-10VPP.4 28.5,14.56 v29.26,14.56 | v54.3,27.13 54.3,15.27 v53.59,14.56 | 55.79,34.52 C58.1 R28.2 54.6,34.39 U4.13
  Bottom 0.406: v53.59,14.56 v29.26,14.56 | v54.3,27.13 54.3,33.4 v55.27,34.37
N$46
  Top 0.254: U5.1 3.41,26.18 R32.2
N$47
  Top 0.406: U12.3 R56.1 R55.2
N$48
  Top 0.254: PCM5101.18 37.6,22 C41.2 36.63,22.11 C2.+
N$49
  Top 0.406: R36.1 13.45,29.71 MB14F.DCPLUS
N$50
  Top 0.305: PCM5101.7 47.58,24.6 R50.2
N$51
  Top 0.305: PCM5101.4 46.26,22.65 47.37,21.54 C49.2
N$52
  Top 0.305: PCM5101.2 46.24,21.35 46.74,20.85 48.34,20.85 48.49,21.01 48.49,21.53 C49.1
N$53
  Top 0.406: C55.1 79.44,37.84 U12.1
N$54
  Top 0.406: MIDI_IN.RIGHT/RING 28.04,39.22 27.38,38.56 24.54,38.56 22.3,36.32 16.08,36.32 14.79,35.03 MB14F.AC1
N$55
  Top 0.406: MIDI_IN.LEFT/TIP 31.68,41.61 27.58,37.52 24.66,37.52 22.71,35.56 16.82,35.56 16.38,35.13 16.38,33.06 MB14F.AC2
N$56
  Top 0.305: D6.C 84.06,36.38 R60.2 84.06,34.79 83.77,34.49 82.19,34.49 U12.4
N$57
  Top 0.406: U15.1 14.38,28.12 D13.- R36.2
N$58  (via drill 0.3)
  Top 0.406: R37.1 v77.8,21.34
  Bottom 0.406: MIDI_OUT.LEFT/TIP 35.99,53.29 36.88,54.18 39.7,54.18 40.74,53.14 44.58,53.14 45.87,54.43 50.6,54.43 52.17,52.86 55.55,52.86 57.15,54.46 59.54,54.46 60.71,53.29 81.18,53.29 84.96,49.51 84.96,23.37 82.93,21.34 v77.8,21.34
N$59  (via drill 0.3)
  Top 0.406: MIDI_OUT.RIGHT/RING 31.68,51.31 34.44,54.08 39.75,54.08 41.05,52.78 44.42,52.78 45.97,54.33 50.83,54.33 52.48,52.68 55.52,52.68 57.2,54.36 60.22,54.36 61.39,53.19 71.78,53.19 72.57,52.4 85.83,52.4 v85.85,52.43 | R38.1 v89.53,34.93
  Bottom 0.406: v89.53,34.93 93.22,38.61 93.22,45.06 v85.85,52.43
N$60  (via drill 0.3)
  Top 0.406: R18.1 U6.3 63.99,37.53 v63.98,37.52 | C29.2 59.09,37.44 R19.2 59.94,38.08 | 59.94,38.08 60.38,38.51 v61.67,38.51 | 59.84,37.39 59.84,37.97 | 59.84,37.97 59.94,38.08 | 59.84,37.97 59.54,37.67 58.83,37.67
  Top 0.61: 58.67,37.39 59.84,37.39
  Bottom 0.406: v61.67,38.51 62.99,38.51 v63.98,37.52
N$61
  Top 0.254: 52.45,35.61 52.5,35.66 U4.14
  Top 0.406: R64.2 49.34,36.13 49.84,35.64 52.43,35.64 52.45,35.61 | U4.14 54.5,35.66 R28.1 C58.2
N$63
  Top 0.406: C57.2 R22.1 54.55,29.08 R63.2 54.52,28.04 U4.8
N$67
  Top 0.254: U1.35 25.92,30.55 25.63,30.84 25.63,33.34 R75.1
N$68
  Top 0.254: U1.33 26.92,32.05 27.96,33.1 R76.1
N$69
  Top 0.406: C63.+ R73.2
N$70
  Top 0.406: R74.2 32.7,12.09 C64.+
N$75
  Top 0.305: SD1.1 88.51,45.85 R39.1
N$76
  Top 0.254: U1.32 27.42,31.94 28.98,33.5 R77.1
N$77
  Top 0.305: SD1.8 87.62,38.15 R43.1
N$78
  Top 0.254: U1.31 27.92,31.73 30.25,34.06 R78.1
N$79
  Top 0.254: U1.30 28.42,31.32 30.15,33.05 R79.1
N$80
  Top 0.254: U1.29 28.92,30.93 30.02,32.03 R80.1
N$81
  Top 0.254: U1.28 29.42,30.61 29.82,31.01 R81.1
N$82
  Top 0.254: U1.4 26.92,19.19 R82.1
N$83
  Top 0.254: U1.5 27.42,18.62 R83.1
N$84
  Top 0.254: U1.6 27.92,19.1 28.37,18.64 R84.1
N$85
  Top 0.254: U1.3 26.42,19.56 26.14,19.28 25.43,19.28 25.27,19.13 R85.1
N$86
  Top 0.254: U1.12 30.92,20.49 32.61,18.8 32.61,18.42 33.17,17.86 R86.1
N$87
  Top 0.254: R87.1 32.35,20.85 U1.13
N$88
  Top 0.254: U1.14 33.42,22.57 33.98,22 R88.1
N$89
  Top 0.254: U1.11 30.42,21.73 30.66,21.97 31.01,21.97 31.7,21.29 31.7,20.49 R89.1
OUTL
  Top 0.305: PCM5101.6 46.87,23.95 47.32,23.5 R51.2
RESET  (via drill 0.3)
  Top 0.305: 88.23,11.49 v88.21,11.51
  Top 0.61: RST.2 88.23,11.49 87.24,11.49 Q2.3 | v95.89,20.41 U2.3 95.89,33.95 C36.2 R47.1
  Bottom 0.61: v95.89,20.41 95.89,19.18 v88.21,11.51
RIN  (via drill 0.3)
  Top 0.406: v52.88,27.15 52.88,16.46 v52.32,15.9 | v31.5,15.9 31.11,15.52 D15.2 30.33,15.77 29.53,15.77 C60.2 27.1,15.86 R1.2
  Bottom 0.406: v52.32,15.9 v31.5,15.9 | LINE_IN.RIGHT/RING 39.82,41.61 42.09,39.35 42.11,39.35 42.19,39.27 51.41,39.27 53.19,41.05 54.61,41.05 56.82,38.66 56.84,37.14 56.84,37.01 55.63,35.79 54.59,35.79 52.88,34.09 v52.88,27.15
RINX
  Top 0.254: U1.48 23.99,19.25 C44.+
RINX_ADC
  Top 0.406: R74.1 C66.2
ROUT  (via drill 0.3)
  Top 0.406: v48.28,36.81 48.45,36.97 R64.1
  Bottom 0.406: LINE_OUT.RIGHT/RING 39.04,46.81 37.59,45.37 37.59,37.26 38.3,36.55 48.03,36.55 v48.28,36.81
ROUT_2V
  Top 0.305: R50.1 48.6,24.46 C51.2 49.9,24.75 50.55,25.4 50.55,32.23 51.44,33.12 U4.12
RTS  (1 unrouted)
  Top 0.305: R9.2 Q2.2 | HOST.6 83.16,9.63 83.72,10.19 83.72,10.54 83.67,10.59
RXD/IO44  (via drill 0.3)
  Top 0.305: U2.36 93.34,15.75 92.48,16.61 v84.23,16.61
  Bottom 0.305: v84.23,16.61 77.93,16.61 HOST.4
SPDIFIN_SIGNAL  (via drill 0.3)
  Top 0.254: 25.63,35.78 R65.1
  Top 0.406: SPDIF_IN.LEFT/TIP 55.49,39.28 40.64,39.28 40.06,38.53 35.48,38.53 33.3,36.35 26.18,36.35 R65.1 | C1.2 v23.27,31.95 D16.2 | v25.63,35.15 25.63,35.78
  Bottom 0.406: v23.27,31.95 23.27,32.79 v25.63,35.15
SPDIFOUT_SIGNAL  (via drill 0.3)
  Top 0.406: SPDIF_OUT.LEFT/TIP 57.99,48.82 55.88,46.71 55.88,43.82 54.23,42.16 v54.23,40.23 | v52.17,27.15 52.17,17.07 v51.77,16.66 | R3.2 36.47,19.55 v36.47,16.66
  Bottom 0.406: v54.23,40.23 55.98,38.48 55.98,37.26 55.22,36.5 54.23,36.5 52.17,34.44 v52.17,27.15 | v36.47,16.66 v51.77,16.66
SPI0_CS0  (via drill 0.3)
  Top 0.305: SD1.2 88.48,44.75 R40.1 D12.1 | U2.18 v86.26,26.42 | D12.1 87.8,43.4 | v88.29,42.85 88.28,42.86 D12.1
  Bottom 0.305: v86.26,26.42 86.26,42.44 86.67,42.85 v88.29,42.85
SPI0_MISO  (via drill 0.3)
  Top 0.305: 88.04,39.25 v87.88,39.25 | v87.88,39.25 SD1.7 | U2.21 v87.88,22.61 | D12.6 87.88,40.97 v87.88,39.25 | R42.1 87.44,38.81 v87.88,39.25
  Bottom 0.305: v87.88,22.61 v87.88,39.25
SPI0_MOSI  (via drill 0.3)
  Top 0.305: U2.19 v85.65,25.15 | 90.97,43.64 SD1.3 90.79,43.46 v88.88,43.46
  Top 0.406: D12.3 v85.65,42.86 85.75,42.96 R41.1
  Bottom 0.305: v85.65,25.15 v85.65,42.86 86.25,43.46 v88.88,43.46
SPI0_SCK  (via drill 0.3)
  Top 0.305: R44.1 87.05,40.02 87.05,40.44 | v89.99,41.43 SD1.5 | U2.20 v87.1,23.88 | 87.05,40.44 D12.5 | v87.1,40.46 87.07,40.46 87.05,40.44
  Bottom 0.305: v87.1,23.88 v87.1,40.46 88.06,41.43 v89.99,41.43
TXD/IO43  (via drill 0.3)
  Top 0.305: U2.37 94.62,15.52 92.89,17.25 v83.74,17.25
  Bottom 0.305: HOST.3 v83.74,17.25
USB_D+
  Top 0.279: 66.2,48.44 USB.B6 66.2,51.3 | USB.A6 67.2,51.34
  Top 0.305: 66.2,48.44 R46.1 | 67.2,51.34 67.03,51.51 66.42,51.51 66.2,51.3
USB_D-
  Top 0.254: 67.72,49.66 67.39,49.33 67.39,49.3 67.69,49
  Top 0.279: USB.B7 67.7,49.33 | USB.A7 66.7,49.48
  Top 0.305: R45.1 67.7,48.29 67.7,49.33 67.39,49.33 66.85,49.33 66.7,49.48
VNEG
  Top 0.305: PCM5101.5 46.6,23.3 47.37,22.53 C48.2
VPWR  (1 unrouted)
  Top 0.406: R14.1 66.73,38.81 67.21,38.33 | 65.08,38.71 65.08,39.4 | 65.08,39.4 64.67,39.8 | 65.08,39.4 65.56,38.91 66.6,38.91
  Top 1.016: C56.1 69.95,44.32 69.52,43.89 | 66.04,39.37 66.17,39.37 67.21,38.33 67.56,37.97 69.11,37.97 69.14,38 69.24,38 | 69.32,38 69.39,38 69.42,38.02 69.34,38.02 69.32,38 | 69.32,38 69.24,38 | 69.24,38 69.16,37.92 69.14,37.92 69.11,37.9 | L3.P$1 69.29,38.05 69.24,38
  Top 1.27: D2.C 69.52,43.89 D14.C 66.75,43.89 66.04,43.18 66.04,42.27 | 66.04,40.72 66.04,39.37 64.67,40.74 | D1.C 65.94,40.82 66.04,40.72 | 64.16,40.87 64.64,40.87 66.04,42.27 | 66.04,42.27 66.04,40.72
XTI
  Top 0.254: U1.39 23.07,26.57 22.73,26.9 22.73,27.75 21.64,28.85 T1.3

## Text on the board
tPlace: GNG | 3V3 | 3V3/IN | SCL | SDA | 3V3 | GND | 5V/IN | + | A12V | + | A5V | + | + | A-12V | + | A3V3 | 3V3 | + | + | + | + | + | 12V/IN | GND | + | NC | GNG | GNG | GNG | 12V_IN | TXD | RXD | 12V_IN | DTR | + | GNG | GNG | GNG | NC | + | + | RTS
bPlace: OUT2 | OUT | OUT | OUT | MIDIIN/ | LINEIN/ | CVIN/ | SPDIFIN/ | CVIN/ | OUT1 | AmyBoard | V1.4
Measures: Units: Inches | Units: Inches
